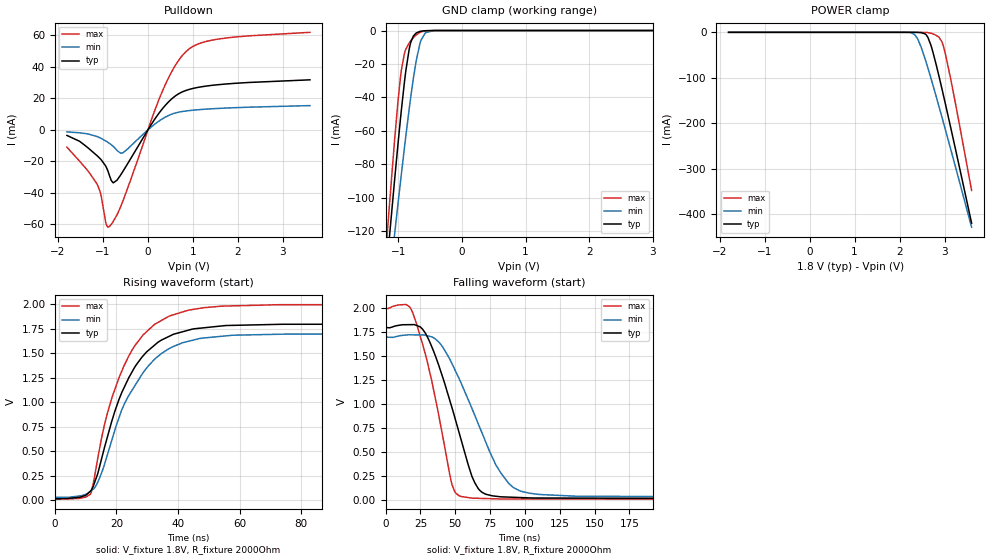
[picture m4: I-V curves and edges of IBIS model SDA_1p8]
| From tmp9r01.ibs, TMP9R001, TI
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|   Model
[Model]   SDA_1p8
Model_type   I/O_open_drain
Polarity   Non-Inverting
Enable   Active-Low
Vinl = 0.54
Vinh = 1.26
Vmeas = 0.9
Vref = 1.8
Cref = 1pF
Rref = 2000
|   typ   min   max
C_comp   1.538pF   1.417pF   1.633pF
[Voltage Range]   1.8   1.7   2
[Temperature Range]   25   125   -40
[Pullup Reference]   1.8   1.7   2
[Pulldown Reference]   0   -0   0
[Power Clamp Reference]   1.8   1.7   2
[GND Clamp Reference]   0   0   0
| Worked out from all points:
|   slope of the pulldown table from 0 to 0.27 V, typ, clamps not added: 23.5 ohm
|   GND clamp passes 1 mA (typ) near -0.69 V on its own axis
|   falling waveform, V_fixture 1.8V, R_fixture 2000Ohm: 20-80 % time 22ns typ, 29.8ns min, 17.3ns max; typ from 1.8 V to 0.019 V
|   rising waveform, V_fixture 1.8V, R_fixture 2000Ohm: 20-80 % time 13.1ns typ, 14.1ns min, 12.7ns max; typ from 0.019 V to 1.8 V
[Pulldown]
|   Voltage   I(typ)   I(min)   I(max)
-1.8V     -3.53mA    -1.303mA   -10.99mA
-1.13V    -16.37mA   -4.247mA   -34.33mA
-1.039V   -18.99mA   -5.437mA   -41.93mA
-930.6mV  -23.37mA   -7.176mA   -59.45mA
-882mV    -26.65mA   -8.063mA   -61.69mA
-774mV    -33.54mA   -10.4mA    -58.17mA
-687.6mV  -31.91mA   -12.95mA   -53.87mA
-547.2mV  -25.93mA   -14.39mA   -44.43mA
311.4mV   13.01mA    6.814mA    23.84mA
840.6mV   24.94mA    11.94mA    49.48mA
1.521V    28.51mA    13.52mA    57.35mA
3.6V      31.71mA    15.37mA    61.83mA
[GND Clamp]
|   Voltage   I(typ)   I(min)   I(max)
-1.8V     -419.3mA   -391mA     -456.2mA
-1.174V   -138.2mA   -162.4mA   -121.6mA
-1.147V   -126.5mA   -152.9mA   -108mA
-1.06V    -90.17mA   -122.7mA   -66.3mA
-952.2mV  -47.65mA   -85.98mA   -23.78mA
-903.6mV  -30.76mA   -70.08mA   -13.64mA
-828mV    -10.91mA   -46.61mA   -7.385mA
-720mV    -1.508mA   -18.24mA   -2.658mA
-644.4mV  -391uA     -5.85mA    -857.3uA
-574.2mV  -95.25uA   -1.285mA   -202.3uA
-444.6mV  -4.546uA   -40.12uA   -6.774uA
3.6V      0A         0A         0A
[POWER Clamp]
|   Voltage   I(typ)   I(min)   I(max)
-1.8V     0A         0A         0A
2.239V    -3.988uA   -527.7uA   -21.99nA
2.336V    -41.66uA   -5.03mA    -192.1nA
2.401V    -167.4uA   -14.41mA   -1.726uA
2.569V    -3.641mA   -58.99mA   -177.9uA
2.628V    -10.91mA   -78mA      -631.8uA
2.714V    -34.32mA   -106.9mA   -2.48mA
2.871V    -94.64mA   -161.5mA   -10.22mA
2.941V    -124.2mA   -186.5mA   -20.83mA
2.979V    -140.5mA   -200.1mA   -32.4mA
3.141V    -211.7mA   -258.8mA   -105.2mA
3.6V      -419.3mA   -428.2mA   -347.4mA
[Ramp]
R_load = 2000
|   typ   min   max
dV/dt_r   1.06867/1.29946e-08   1.00015/1.40492e-08   1.19298/1.26531e-08
dV/dt_f   1.06863/2.19602e-08   0.999937/2.96481e-08   1.19297/1.72993e-08
[Falling Waveform]
V_fixture = 1.8V
V_fixture_min = 1.7V
V_fixture_max = 2V
R_fixture = 2000Ohm
C_fixture = 0F
|   Time   V(typ)   V(min)   V(max)
0s        1.8V       1.7V       2V
14.48ns   1.829V     1.722V     2.04V
19.63ns   1.83V      1.724V     1.949V
32.04ns   1.639V     1.707V     1.315V
47.3ns    983.2mV    1.435V     186.9mV
52.66ns   711.7mV    1.272V     50.46mV
67.28ns   109.8mV    771.4mV    22.05mV
82.66ns   38.01mV    287.7mV    15.81mV
96.73ns   30.26mV    98.57mV    15.54mV
300ns     18.95mV    33.44mV    11.72mV
[Rising Waveform]
V_fixture = 1.8V
V_fixture_min = 1.7V
V_fixture_max = 2V
R_fixture = 2000Ohm
C_fixture = 0F
|   Time   V(typ)   V(min)   V(max)
0s        18.88mV    33.08mV    11.71mV
11.54ns   94.01mV    92.4mV     63.05mV
13.96ns   276.3mV    187.3mV    431.7mV
17.26ns   669.8mV    486.4mV    911.3mV
20.84ns   1.031V     844.6mV    1.252V
24.18ns   1.262V     1.08V      1.485V
32.94ns   1.6V       1.457V     1.807V
43.37ns   1.738V     1.624V     1.942V
75.78ns   1.798V     1.698V     1.998V
300ns     1.8V       1.7V       2V
